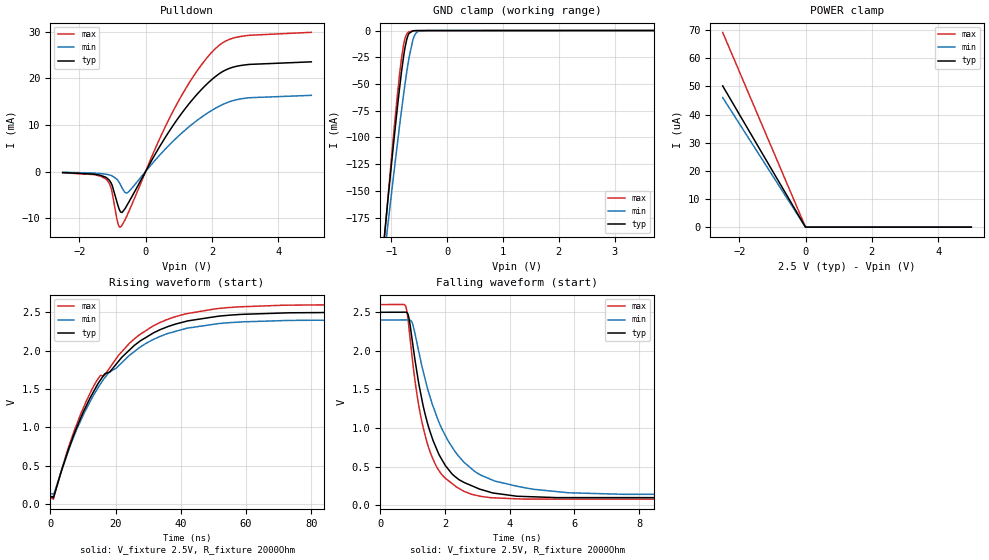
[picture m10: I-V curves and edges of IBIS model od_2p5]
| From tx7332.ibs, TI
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|   od_2p5 Model
[Model]   od_2p5
Model_type   Open_drain
Polarity   Inverting
Vmeas = 1.25
Vref = 2.5
Cref = 2pF
Rref = 2000
|   typ   min   max
C_comp   6.218pF   6.161pF   6.363pF
| Where Nom  PVT is Nominal Process, 2.5V, 27C
|   Fast PVT is Strong Process,  2.6V, 0C
|   Slow PVT is Weak Process,   2.4V, 100C
[Voltage Range]   2.5   2.4   2.6
|Junction Temperature
[Temperature Range]   27   100   0
[Pullup Reference]   2.5   2.4   2.6
[Pulldown Reference]   0   0   0
[Power Clamp Reference]   2.5   2.4   2.6
[GND Clamp Reference]   0   0   0
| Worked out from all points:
|   slope of the pulldown table from 0 to 0.375 V, typ, clamps not added: 78.9 ohm
|   GND clamp passes 1 mA (typ) near -0.64 V on its own axis
|   falling waveform, V_fixture 2.5V, R_fixture 2000Ohm: 20-80 % time 899ps typ, 1.31ns min, 709ps max; typ from 2.5 V to 0.095 V
|   rising waveform, V_fixture 2.5V, R_fixture 2000Ohm: 20-80 % time 20ns typ, 19.9ns min, 19.9ns max; typ from 0.095 V to 2.5 V
[Pulldown]
|   Voltage   I(typ)   I(min)   I(max)
-2.5V     -224.6uA   -150.7uA   -258.4uA
-1.18V    -1.321mA   -600.7uA   -1.715mA
-1.045V   -2.391mA   -839.5uA   -3.469mA
-857.5mV  -6.703mA   -1.713mA   -10.49mA
-760mV    -8.603mA   -2.822mA   -11.92mA
-617.5mV  -7.945mA   -4.53mA    -10.32mA
-512.5mV  -6.646mA   -4.36mA    -8.696mA
852.5mV   10.13mA    6.673mA    13.27mA
1.468V    15.89mA    10.51mA    20.71mA
2.007V    19.81mA    13.17mA    25.69mA
2.848V    22.74mA    15.57mA    28.98mA
5V        23.55mA    16.36mA    29.89mA
[GND Clamp]
|   Voltage   I(typ)   I(min)   I(max)
-2.5V     -962.2mA   -868.7mA   -1.072A
-1.15V    -204.8mA   -221.4mA   -209.4mA
-1.067V   -160.6mA   -183.4mA   -159.2mA
-895mV    -72.68mA   -106.4mA   -60.92mA
-820mV    -38.85mA   -74.89mA   -26.01mA
-760mV    -16.98mA   -51.27mA   -8.027mA
-722.5mV  -7.701mA   -37.69mA   -2.979mA
-685mV    -2.699mA   -25.5mA    -1.13mA
-617.5mV  -319.3uA   -9.096mA   -304.1uA
-587.5mV  -148.9uA   -4.819mA   -194.5uA
-467.5mV  -60.67uA   -224uA     -88.69uA
5V        0A         0A         0A
[POWER Clamp]
|   Voltage   I(typ)   I(min)   I(max)
-2.5V     50.19uA    46.06uA    69.21uA
-10mV     153.1nA    137.2nA    229.4nA
-2.5mV    2.535nA    68.59nA    21.73nA
5V        0A         0A         0A
[Ramp]
R_load = 2000
|   typ   min   max
dV/dt_r   1.44297/1.99406e-08   1.35797/1.98487e-08   1.5141/1.98942e-08
dV/dt_f   1.44297/8.93769e-10   1.35797/1.30492e-09   1.5141/7.06847e-10
[Falling Waveform]
V_fixture = 2.5V
V_fixture_min = 2.4V
V_fixture_max = 2.6V
R_fixture = 2000Ohm
C_fixture = 0F
|   Time   V(typ)   V(min)   V(max)
0s        2.5V       2.4V       2.6V
783.5ps   2.501V     2.401V     2.584V
876.7ps   2.443V     2.401V     2.334V
992.8ps   2.12V      2.357V     1.886V
1.28ns    1.384V     1.815V     1.094V
1.549ns   940.9mV    1.39V      680.4mV
1.857ns   625.8mV    1.034V     422.4mV
2.911ns   237.5mV    440.6mV    133.7mV
4.462ns   113.1mV    227.3mV    79.26mV
300ns     95.04mV    136.7mV    76.49mV
[Rising Waveform]
V_fixture = 2.5V
V_fixture_min = 2.4V
V_fixture_max = 2.6V
R_fixture = 2000Ohm
C_fixture = 0F
|   Time   V(typ)   V(min)   V(max)
0s        95.04mV    136.7mV    76.49mV
914.7ps   83.34mV    127.2mV    59.02mV
5.422ns   687.9mV    674.2mV    718.2mV
9.44ns    1.131V     1.096V     1.183V
15.23ns   1.606V     1.554V     1.667V
16.54ns   1.688V     1.636V     1.673V
27.13ns   2.111V     2.031V     2.199V
41.42ns   2.378V     2.285V     2.478V
71.4ns    2.489V     2.39V      2.591V
300ns     2.5V       2.4V       2.6V
